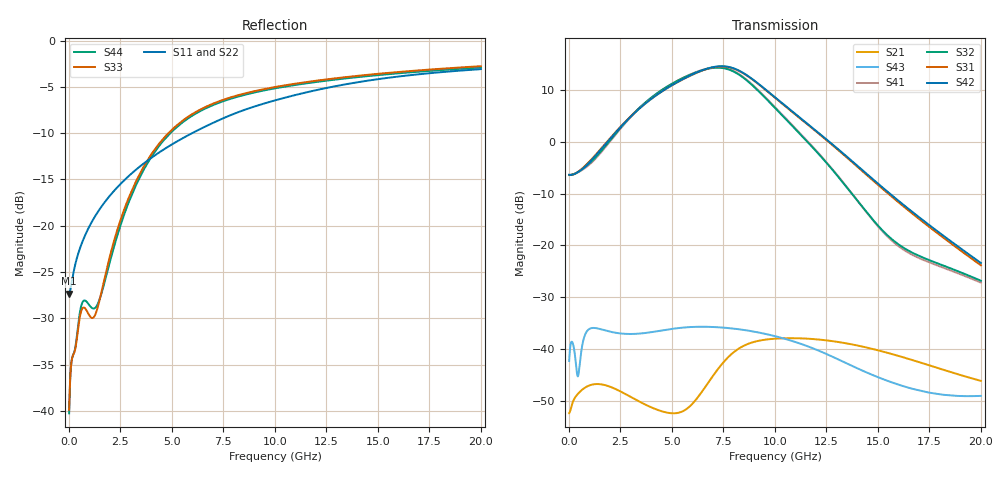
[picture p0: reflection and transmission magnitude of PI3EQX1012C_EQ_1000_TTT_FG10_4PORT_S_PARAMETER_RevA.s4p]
! NPort=4 DATA=2000 NOISE=0 GROUPDELAY=0 COMPLEX_DATAFORMAT=POLAR
! NumOfBlock=1 NumOfParam=0
! .MODEL Smodel S TSTONEFILE=PI3EQX1012C_EQ_1000_TTT_FG10_4PORT_S_PARAMETER_RevA.s4p TYPE=S
!  -- The above .MODEL line can be used for the S element in the netlist.
! The s parameter is extracted from the linear redriver, it is not bi-directional; only s(4,1)s(4,2) and s(3,1)s(3,2)
! should be the insertion loss
!Port definition:
!Port1 = input+
!Port2 = input-
!Port3 = output+
!Port4 = output-
# Hz S MA R  50
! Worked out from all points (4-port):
!   2000 points, 10 MHz to 20 GHz, reference 50 ohm
!   strongest paths, dB at 10 MHz, 5.01 GHz, 10.01 GHz, 15.01 GHz, 20 GHz:
!     S42: -6.4, 11.0, 8.6, -8.1, -23.4
!     S31: -6.4, 10.9, 8.5, -8.3, -23.9
!     S32: -6.4, 11.2, 6.5, -16.2, -26.9
!     S41: -6.4, 11.2, 6.7, -16.4, -27.2
!     S43: -42.4, -36.2, -37.6, -45.5, -49.1
!     S21: -52.4, -52.5, -38.1, -40.3, -46.2
!   lowest |S11| = -27.3 dB at 10 MHz (marker M1), VSWR 1.09, Z = 45.9 - j0.123 ohm
!   |S11| at or under -10 dB: start of sweep to 5.983 GHz
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1e7  0.04301 -178.2  0.002379 1.5  0.0008102 -0.5  0.0008039 -0.5
     0.002388 1.5  0.04109 -178.1  0.000927 -0.5  0.0009197 -0.5
     0.4784 -0.1  0.4775 -180.0  0.01016 -4.0  0.007598 -25.7
     0.4771 180.0  0.4794 -0.1  0.007615 -25.8  0.009722 -4.0
4.08e9  0.236 -124.3  0.002699 0.1  0.0003831 -56.7  0.0003813 -57.1
        0.002673 0.2  0.2396 -123.2  0.0004355 -57.4  0.0004334 -57.8
        2.674 -61.3  2.751 128.3  0.2506 -83.4  0.01357 34.0
        2.737 129.0  2.672 -59.7  0.01455 31.0  0.2427 -83.1
5.68e9  0.3036 -123.7  0.002663 42.0  0.0002805 -58.4  0.0002793 -59.3
        0.002592 40.2  0.3085 -123.0  0.0003181 -59.4  0.0003168 -60.3
        4.154 -128.3  4.268 61.1  0.3806 -98.8  0.01634 10.6
        4.284 61.4  4.172 -126.4  0.0161 7.8  0.3729 -98.6
6.96e9  0.3577 -124.3  0.005623 60.5  0.0002413 -56.0  0.0002393 -57.3
        0.005353 61.0  0.3632 -123.8  0.0002723 -57.2  0.0002702 -58.5
        5.221 168.0  5.165 -3.0  0.4546 -108.9  0.01674 -9.5
        5.21 -3.1  5.252 170.1  0.01624 -10.5  0.4464 -108.8
8.09e9  0.4053 -125.7  0.009855 43.2  0.0002247 -54.3  0.0002217 -55.8
        0.009557 44.6  0.4113 -125.2  0.0002519 -55.6  0.0002487 -57.1
        5.014 103.3  4.666 -67.7  0.5023 -115.8  0.01593 -25.1
        4.724 -68.1  5.048 105.6  0.01558 -25.4  0.4938 -115.7
9.45e9  0.4561 -128.0  0.01237 15.2  0.0002145 -53.8  0.0002104 -55.4
        0.01218 16.5  0.463 -127.6  0.0002387 -55.0  0.0002344 -56.6
        3.293 33.8  2.762 -135.9  0.546 -122.1  0.01432 -41.4
        2.806 -136.9  3.318 36.4  0.01404 -42.0  0.5372 -122.0
2e10  0.7009 -144.6  0.004927 -72.7  0.0001465 -72.3  0.0001413 -73.8
      0.004895 -71.6  0.716 -144.4  0.0001624 -72.1  0.0001567 -73.8
      0.06403 105.0  0.04543 31.2  0.7272 -143.5  0.003585 -51.6
      0.04352 29.3  0.06745 109.6  0.003504 -48.9  0.7152 -143.3
